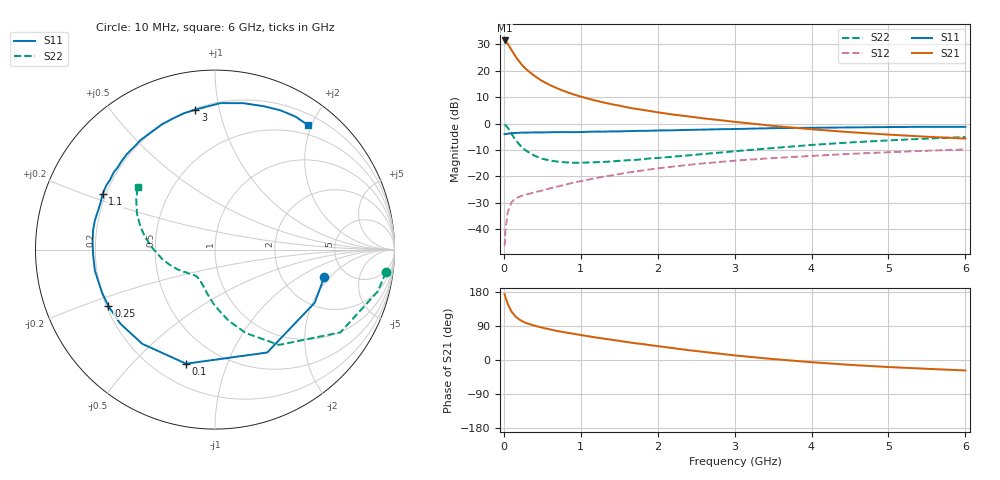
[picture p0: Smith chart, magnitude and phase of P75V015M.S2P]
! SIEMENS Small Signal Semiconductors
! BFP196
! Si NPN RF Bipolar Junction Transistor in SOT143
! VCE = 5 V  IC = 15 mA
! Common Emitter S-Parameters:  May  1996
# GHz  S  MA  R  50
!  f  S11  S21  S12  S22
! GHz  MAG  ANG  MAG  ANG  MAG  ANG  MAG  ANG
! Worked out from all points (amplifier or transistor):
!   36 points, 10 MHz to 6 GHz, reference 50 ohm
!   highest |S21| = 31.4 dB at 10 MHz (marker M1)
!   |S21| within 3 dB of that: start of sweep to 86.99 MHz
!   unconditionally stable (mu >= 1): 786.6 MHz to 3.37 GHz
!   at 250 MHz: K = 0.50, MSG = 24.4 dB, |S12| = -27.2 dB
!   at 1.4 GHz: K = 1.12, MAG = 11.4 dB, |S12| = -19.6 dB
!   at 6 GHz: K = 0.96, MSG = 2.1 dB, |S12| = -9.8 dB
!   S11 on the Smith chart (normalised r, x): 10 MHz: 3.42, -1.74; 100 MHz: 0.33, -0.73; 250 MHz: 0.21, -0.24; 1.1 GHz: 0.19, +0.22; 3 GHz: 0.21, +0.85; 6 GHz: 0.35, +1.95
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0.01  0.6275 -14.2  37.17 173.7  0.0048 83.5  0.9608 -7.5
0.02  0.6296 -28.0  36.12 165.9  0.0091 78.4  0.9371 -14.3
0.05  0.6429 -63.1  32.3 148.5  0.021 62.7  0.8375 -33.4
0.1  0.6559 -104.2  24.48 127.8  0.0326 48.4  0.6398 -56.1
0.15  0.6632 -127.6  18.66 115.0  0.0383 41.4  0.4953 -69.8
0.2  0.6696 -141.9  14.89 106.9  0.0412 38.9  0.4029 -79.2
0.25  0.6722 -152.0  12.17 101.1  0.0438 37.3  0.3396 -86.2
0.3  0.6735 -159.1  10.33 96.9  0.0458 37.9  0.2998 -91.9
0.4  0.6794 -170.0  7.908 90.6  0.0499 39.6  0.2453 -100.7
0.5  0.6796 -177.3  6.35 85.4  0.0542 41.7  0.2156 -107.1
0.6  0.6837 176.4  5.323 80.7  0.0595 43.6  0.1997 -112.2
0.8  0.6889 166.4  4.019 72.7  0.0699 46.2  0.1846 -120.5
0.9  0.6866 161.8  3.571 69.3  0.0759 47.2  0.1811 -123.5
1.1  0.6984 153.8  2.94 62.6  0.0871 48.7  0.1836 -128.7
1.3  0.7022 146.3  2.492 56.3  0.0992 48.7  0.1881 -133.3
1.6  0.717 136.4  2.028 47.4  0.1176 47.9  0.2019 -139.9
2.2  0.7443 118.7  1.478 31.3  0.1537 43.4  0.2358 -152.1
3  0.7873 98.0  1.077 12.1  0.1984 34.8  0.2992 -170.1
3.5  0.8168 87.9  0.903 2.5  0.2222 29.1  0.3441 179.5
4.5  0.8435 71.3  0.686 -12.8  0.2666 18.0  0.4381 162.3
5.5  0.8662 58.9  0.562 -23.2  0.3057 7.1  0.519 147.7
6  0.8658 53.2  0.52 -27.6  0.324 1.2  0.5551 140.9
